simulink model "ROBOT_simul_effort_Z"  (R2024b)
settings: Solver=VariableStepAuto  StartTime=0.0  StopTime=5  RelTol=1e-3
undefined symbols (not defined in the file): a, ARRIERE_Defaut_sldprt, avant01_Defaut_sldprt, avant02_Defaut_sldprt, avant03_Defaut_sldprt, avant1_Defaut_sldprt, AXE, BASE_Defaut_sldprt, BIELLE, BIELLE_Defaut_sldprt, BRAS_Defaut_sldprt, bras_Defaut_sldprt, C_Realiste_sldprt, CABLE_Defaut_sldprt, cable_Defaut_sldprt, CACHE_Defaut_sldprt, CARTE, carte_Defaut_sldprt, CARTER, carter, CHC, CODEUR_Defaut_sldprt, cruciforme, cylindrique, deg, Drive, Fichiers, Fichiers_Matlab_sujetA, FIXATION, fixation_Defaut_sldprt, H, HEXAGONALE_Defaut_sldprt, joint_Defaut_sldprt, kg, m, M4, M4_Defaut_sldprt, manette1_Defaut_sldprt, manette2_Defaut_sldprt, MATLAB, Matlab, matlab_Defaut_sldprt, mm, modif, MOTEUR_Defaut_sldprt, N, NEZ_Defaut_sldprt, nom, palier, PARALLELOGRAMME_Defaut_sldprt, petite, plaque, rad, Ressort, Rondelle, ROTOR_Defaut_sldprt, s, SET, simple, socle_Defaut_sldprt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
libraries: sm_lib x463, fl_lib x45, nesl_utility x27, simulink x2
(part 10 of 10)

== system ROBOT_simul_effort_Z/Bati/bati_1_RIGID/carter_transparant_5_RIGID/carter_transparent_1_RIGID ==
  ReferenceFrame : sm_lib/Frames and Transforms/Reference Frame
  Solid : sm_lib/Body Elements/File Solid  ExtGeomFileName=/MATLAB Drive/Fichiers_Matlab_sujetA/Fichiers Matlab/STL/carter transparent_Defaut_sldprt.STL  UnitType=Custom  ExtGeomFileUnits=mm  StepReaderType=HEX  ExportConvexHullGeometry=off  InertiaType=Custom  BasedOnType=Density  Density=1000  DensityUnits=kg/(m^3)  Mass=0.056273911834023478  MassUnits=kg  CenterOfMass=[12.60882798450937 60.199925046373778 61.212214588211637]  CenterOfMassUnits=mm  MomentsOfInertia=[58.20868427615801 95.569253812513907 86.337959151344037]  MomentsOfInertiaUnits=kg*mm^2  ProductsOfInertia=[-17.408508514500589 1.3730953848150378 -5.3261234176687369]  ProductsOfInertiaUnits=kg*mm^2  GraphicType=FromGeometry  MarkerShape=Sphere  MarkerSize=10  GraphicVisPropType=SimpleVisualProperties  GraphicDiffuseColor=[0.792156862745098 0.81960784313725488 0.93333333333333335]  GraphicOpacity=1  GraphicSpecularColor=[0.5 0.5 0.5 1.0]  GraphicAmbientColor=[0.15 0.15 0.15 1.0]  GraphicEmissiveColor=[0.0 0.0 0.0 1.0]  GraphicShininess=75  DoExposeReferenceFrame=on  SerializedFrames=<Frames/>
  F : PMIOPort  Side=Left
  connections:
  Solid/RConn1 -- ReferenceFrame/RConn1 -- F/RConn1

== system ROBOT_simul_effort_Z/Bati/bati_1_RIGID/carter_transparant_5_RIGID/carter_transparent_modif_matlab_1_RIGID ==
  ReferenceFrame : sm_lib/Frames and Transforms/Reference Frame
  Solid : sm_lib/Body Elements/File Solid  ExtGeomFileName=/MATLAB Drive/Fichiers_Matlab_sujetA/Fichiers Matlab/STL/carter transparent modif matlab_Defaut_sldprt.STL  UnitType=Custom  ExtGeomFileUnits=mm  StepReaderType=HEX  ExportConvexHullGeometry=off  InertiaType=Custom  BasedOnType=Density  Density=1000  DensityUnits=kg/(m^3)  Mass=0.044889069172440496  MassUnits=kg  CenterOfMass=[-16.380945858412954 64.543634175323007 61.916354268852707]  CenterOfMassUnits=mm  MomentsOfInertia=[48.669303101169348 65.98246777989317 58.974719121474422]  MomentsOfInertiaUnits=kg*mm^2  ProductsOfInertia=[-12.770089995694509 -9.4582724645364351 -6.681394862606262]  ProductsOfInertiaUnits=kg*mm^2  GraphicType=FromGeometry  MarkerShape=Sphere  MarkerSize=10  GraphicVisPropType=SimpleVisualProperties  GraphicDiffuseColor=[0.792156862745098 0.81960784313725488 0.93333333333333335]  GraphicOpacity=1  GraphicSpecularColor=[0.5 0.5 0.5 1.0]  GraphicAmbientColor=[0.15 0.15 0.15 1.0]  GraphicEmissiveColor=[0.0 0.0 0.0 1.0]  GraphicShininess=75  DoExposeReferenceFrame=on  SerializedFrames=<Frames/>
  F : PMIOPort  Side=Left
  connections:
  Solid/RConn1 -- ReferenceFrame/RConn1 -- F/RConn1
